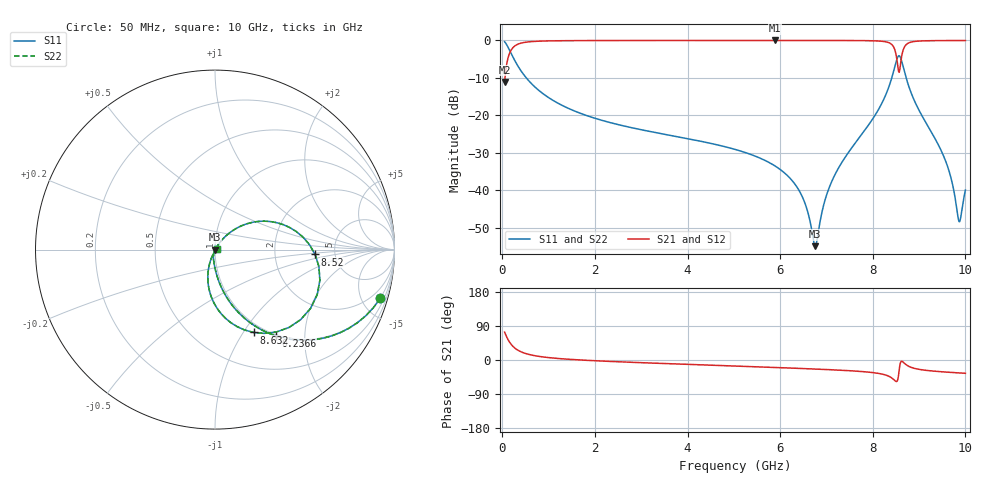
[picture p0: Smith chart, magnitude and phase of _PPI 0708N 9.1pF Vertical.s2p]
! S-Parameter data specifications (vertical orientation):
! Substrate: 40-mil Rogers 3003C, Substrate thickness, H=1.016mm, Dielectric constant, Er=3, Conductor thickness, T_mtl=0.043mm, Loss Tangent, Tand=0.003
! PCB Mounting Pad Footprint: Pad width, PadW=2.54mm , Pad length, PadL=0.51mm , Pad gap, PadG (edge-to-edge)=0.71mm , Reference planes=1.73mm apart
! Created Tue Jan 16 08:46:52 2018
# GHz S MA R 50
! 2 Port Network Data from SP1.SP block
! freq  magS11  angS11  magS21  angS21  magS12  angS12  magS22  angS22
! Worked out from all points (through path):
!   801 points, 50 MHz to 10 GHz, reference 50 ohm
!   highest |S21| = -0.02 dB at 5.896 GHz (marker M1); lowest = -11.1 dB at 50 MHz (marker M2)
!   group delay of S21, straight-line fit = 14.7 ps
!   lowest |S11| = -54.9 dB at 6.754 GHz (marker M3), VSWR 1.00, Z = 50.2 - j0.0913 ohm
!   |S11| at or under -10 dB: 518.7 MHz to 8.41 GHz (7.891 GHz wide, 177 % of centre); 8.721 GHz to end of sweep
!   |S22| runs from -54.9 to -0.4 dB; largest |S21 - S12| = 0
!   S11 on the Smith chart (normalised r, x): 50 MHz: 0.98, -6.81; 236.6 MHz: 0.98, -1.44; 8.52 GHz: 3.51, -0.28; 8.632 GHz: 0.89, -1.11; 10 GHz: 1.02, +0.01
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0.05  0.9602 -16.4  0.2791 73.6  0.2791 73.6  0.9602 -16.4
0.2365625  0.5884 -54.8  0.8083 35.2  0.8083 35.2  0.5884 -54.8
0.6096875  0.2733 -76.3  0.9616 13.7  0.9616 13.7  0.2733 -76.3
1.716625  0.105 -89.9  0.9939 -0.2  0.9939 -0.2  0.105 -89.9
3.370812  0.0581 -98.0  0.9974 -8.8  0.9974 -8.8  0.0581 -98.0
5.025  0.03527 -104.1  0.9981 -15.9  0.9981 -15.9  0.03527 -104.1
5.895625  0.02109 -106.1  0.9982 -19.7  0.9982 -19.7  0.02109 -106.1
6.418  0.009757 -102.9  0.9981 -22.2  0.9981 -22.2  0.009757 -102.9
6.691625  0.002744 -73.9  0.998 -23.5  0.998 -23.5  0.002744 -73.9
6.753813  0.001809 -30.2  0.9979 -23.8  0.9979 -23.8  0.001809 -30.2
6.96525  0.00732 49.2  0.9977 -25.0  0.9977 -25.0  0.00732 49.2
7.151813  0.01481 55.2  0.9973 -26.0  0.9973 -26.0  0.01481 55.2
8.022438  0.09473 51.7  0.9873 -33.5  0.9873 -33.5  0.09473 51.7
8.345812  0.2387 38.0  0.9333 -42.8  0.9333 -42.8  0.2387 38.0
8.45775  0.4043 20.2  0.8 -52.2  0.8 -52.2  0.4043 20.2
8.519937  0.5584 -2.8  0.5622 -56.5  0.5622 -56.5  0.5584 -2.8
8.569688  0.6251 -31.5  0.3752 -27.2  0.3752 -27.2  0.6251 -31.5
8.631875  0.5094 -65.0  0.6505 -3.5  0.6505 -3.5  0.5094 -65.0
8.793563  0.2286 -98.0  0.9356 -17.6  0.9356 -17.6  0.2286 -98.0
9.577125  0.02428 -111.3  0.9949 -31.9  0.9949 -31.9  0.02428 -111.3
9.85075  0.004076 -53.7  0.9958 -34.0  0.9958 -34.0  0.004076 -53.7
10  0.01012 33.5  0.9959 -35.1  0.9959 -35.1  0.01012 33.5
